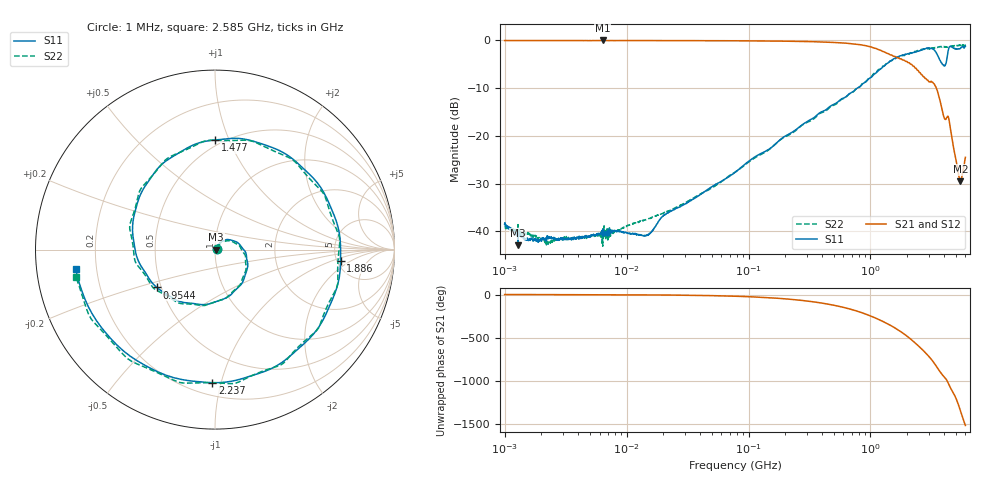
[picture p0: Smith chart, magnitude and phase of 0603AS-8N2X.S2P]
!s-Parameter Generated by FASTRON Sdn. Bhd.
!FASTRON P/N : 0603AS-8N2X
!Keysight Technologies: E5071C_MY46733604_B.14.02
!Date: Mon Dec 04 10:08:45 2023
!Version  :Rev01  Mon Dec 04 10:08:45 2023
!Data & Calibration Information:
!Freq  S11:SOLT2(ON)  S21:SOLT2(ON)  S12:SOLT2(ON)  S22:SOLT2(ON)
!PortZ  Port1:50+j0  Port2:50+j0
!When reading reference impedance value at option line is always used.
! Remarks : This data is being provided solely for informational purposes.
# Hz S dB R 50
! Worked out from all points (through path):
!   1601 points, 1 MHz to 6 GHz, reference 50 ohm
!   highest |S21| = -0.06 dB at 6.378 MHz (marker M1); lowest = -29.5 dB at 5.468 GHz (marker M2)
!   group delay of S21, straight-line fit = 671 ps
!   lowest |S11| = -42.9 dB at 1.288 MHz (marker M3), VSWR 1.01, Z = 50.7 + j0.0518 ohm
!   |S11| at or under -10 dB: start of sweep to 780.9 MHz
!   |S22| runs from -43.1 to -1.0 dB; largest |S21 - S12| = 0.0075
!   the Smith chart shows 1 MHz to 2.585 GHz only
!   S11 on the Smith chart (normalised r, x): 1 MHz: 1.02, +0.01; 954.4 MHz: 0.47, -0.23; 1.477 GHz: 0.46, +0.89; 1.886 GHz: 5.39, -1.30; 2.237 GHz: 0.29, -0.94; 2.585 GHz: 0.12, -0.07
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1000000  -38.43 14.0  -0.08 -0.1  -0.09 -0.2  -38.89 12.1
1287650  -42.92 4.1  -0.08 -0.2  -0.07 -0.2  -38.58 3.7
4277066  -41.40 20.0  -0.09 -1.1  -0.08 -1.1  -41.40 20.6
6378092  -41.05 31.1  -0.06 -1.7  -0.11 -1.8  -43.08 18.7
1.823719e7  -37.94 42.3  -0.09 -4.7  -0.10 -4.6  -36.50 41.8
7.757876e7  -27.65 54.6  -0.13 -19.5  -0.13 -19.5  -27.60 50.9
3.307917e8  -16.47 4.5  -0.31 -82.0  -0.31 -82.0  -16.73 1.5
6.68109e8  -11.24 -75.3  -0.70 -165.1  -0.69 -165.1  -11.26 -75.7
9.544369e8  -8.24 -147.0  -1.28 123.9  -1.28 123.9  -8.07 -144.6
1.414819e9  -4.61 104.7  -2.90 13.4  -2.90 13.4  -4.63 102.2
1.476521e9  -4.28 89.9  -3.09 -0.3  -3.08 -0.4  -4.31 89.2
1.886156e9  -3.07 -5.0  -4.18 -95.9  -4.19 -95.8  -3.24 -6.3
2.23694e9  -2.60 -91.1  -5.42 -178.7  -5.42 -178.6  -2.50 -84.4
2.584893e9  -2.11 -171.9  -7.04 99.8  -7.01 100.0  -2.05 -168.9
3.068351e9  -1.69 83.4  -8.77 -7.3  -8.72 -7.4  -1.86 78.4
3.462469e9  -2.65 -18.5  -10.02 -108.2  -10.00 -108.5  -1.53 -8.8
3.847204e9  -4.84 -125.8  -14.34 159.3  -14.36 158.8  -1.41 -98.9
4.211689e9  -4.14 176.1  -16.21 92.4  -16.24 92.1  -1.49 176.5
4.628987e9  -1.41 95.9  -20.08 -22.3  -20.12 -22.5  -1.25 84.8
5.048685e9  -1.89 23.5  -25.28 -126.5  -25.32 -126.6  -1.18 -6.5
5.468383e9  -1.69 -67.5  -29.53 93.6  -29.57 93.6  -1.02 -96.1
6e9  -1.27 168.7  -24.50 -72.6  -24.51 -72.4  -1.22 156.9
